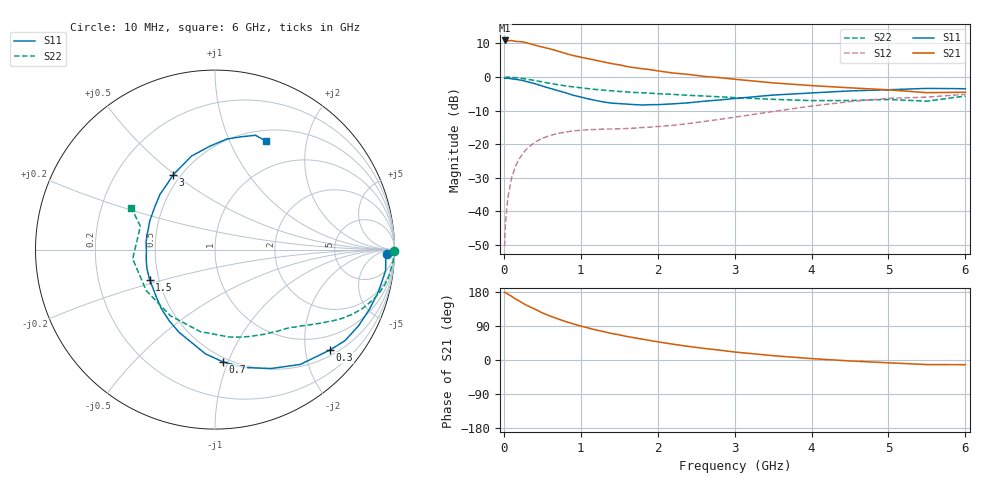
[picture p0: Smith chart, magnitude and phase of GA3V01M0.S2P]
! Infineon Technologies  Discrete & RF Semiconductors
! BF775
! Si NPN RF Bipolar Junction Transistor in SOT23
! VCE = 3 V  IC = 1 mA
! Common Emitter S-Parameters:  May  1996
# GHz  S  MA  R  50
!  f  S11  S21  S12  S22
! GHz  MAG  ANG  MAG  ANG  MAG  ANG  MAG  ANG
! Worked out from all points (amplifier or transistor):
!   36 points, 10 MHz to 6 GHz, reference 50 ohm
!   highest |S21| = 10.9 dB at 10 MHz (marker M1)
!   |S21| within 3 dB of that: start of sweep to 676 MHz
!   unconditionally stable (mu >= 1): 1.416 GHz to 4.324 GHz; 5 GHz to end of sweep
!   at 250 MHz: K = 0.20, MSG = 16.6 dB, |S12| = -22.7 dB
!   at 1.4 GHz: K = 0.99, MSG = 9.8 dB, |S12| = -15.5 dB
!   at 6 GHz: K = 1.04, MAG = -0.8 dB, |S12| = -5.2 dB
!   S11 on the Smith chart (normalised r, x): 10 MHz: 35, -19; 300 MHz: 0.63, -2.54; 700 MHz: 0.47, -0.96; 1.5 GHz: 0.44, -0.18; 3 GHz: 0.46, +0.49; 6 GHz: 0.63, +1.38
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0.01  0.9567 -1.4  3.505 179.2  0.003 90.5  0.9999 -0.6
0.02  0.9522 -2.8  3.457 177.5  0.0063 89.0  0.9864 -1.2
0.05  0.9579 -7.0  3.457 174.1  0.0153 84.8  0.9959 -3.1
0.1  0.9407 -14.3  3.498 168.1  0.0312 81.4  0.9869 -6.1
0.15  0.9227 -21.1  3.397 161.2  0.046 76.7  0.9782 -9.3
0.25  0.8843 -35.0  3.341 149.6  0.0733 68.6  0.9467 -14.7
0.3  0.8513 -41.0  3.223 144.0  0.0851 64.8  0.9265 -17.3
0.5  0.7327 -64.7  2.794 124.4  0.1219 52.6  0.8445 -25.3
0.6  0.6771 -76.0  2.627 116.1  0.1344 47.6  0.804 -28.5
0.7  0.6273 -85.9  2.437 108.7  0.1434 43.8  0.7677 -31.1
0.9  0.5345 -104.0  2.09 95.5  0.157 37.8  0.7128 -35.2
1.1  0.4714 -122.8  1.871 84.4  0.1636 34.4  0.6689 -38.9
1.2  0.4451 -132.0  1.769 79.1  0.1651 33.0  0.6512 -40.6
1.5  0.4008 -155.3  1.518 66.4  0.1691 32.3  0.6082 -45.4
1.9  0.3863 174.0  1.287 51.4  0.1782 34.5  0.5727 -52.6
2.2  0.3975 155.9  1.146 41.7  0.1903 37.2  0.55 -58.7
3  0.4775 119.2  0.926 21.1  0.2516 41.7  0.493 -81.0
3.5  0.5374 104.1  0.817 11.4  0.3057 40.0  0.4642 -100.1
4.5  0.6201 83.8  0.689 -2.5  0.4296 28.9  0.4459 -149.0
5  0.6454 76.9  0.643 -7.4  0.4804 20.9  0.4617 -173.5
5.5  0.6757 70.5  0.584 -12.0  0.5009 11.9  0.4358 162.6
6  0.6682 64.7  0.592 -12.3  0.5507 7.3  0.5199 153.6
